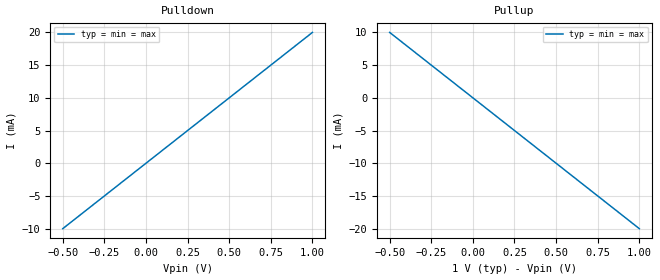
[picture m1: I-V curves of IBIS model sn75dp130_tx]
[IBIS Ver]   5.0
[File Name]  sn75dp130.ibs
[File Rev]   1.0
[Component]  sn75dp130
[Manufacturer] Texas Instruments Incorporated
[Package]
R_pkg  0.0   NA   NA
L_pkg  0.0   NA   NA
C_pkg  0.0   NA   NA
[Pin]   signal_name   model_name   R_pin L_pin  C_pin
1p   Tx_p   sn75dp130_tx
1n   Tx_n   sn75dp130_tx
2p   Rx_p   sn75dp130_rx
2n   Rx_n   sn75dp130_rx
[Diff_Pin] inv_pin vdiff tdelay_typ tdelay_min tdelay_max
2p   2n   NA   NA   NA   NA
1p   1n   NA   NA   NA   NA
[Repeater Pin]
2p 1p
[Model] sn75dp130_rx
Model_type Input
C_comp 0p 0p 0p
Vinl = 0.3
Vinh = 0.7
[Temperature_Range] 25 125 0
[Voltage Range] 1.0 1.0 1.0
[Algorithmic Model]
|Executable Windows_VisualC++ExpressEdition9.0.30729_32 IdealRx.dll IdealRx.ami
Executable Windows_cl15.00.30729.01_32 RX_SN75DP130.dll RX_SN75DP130.ami
[End Algorithmic Model]
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| Models and submodels in the file (2): sn75dp130_tx (Output), sn75dp130_rx (Input)
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[Model] sn75dp130_tx
Model_type Output
C_comp 0p 0p 0p
Cref = 0
Vref = 0.5
Rref = 50
Vmeas = 0.5
[Temperature_Range] 25 125 0
[Voltage Range] 1 1 1
[Algorithmic Model]
|Executable Windows_VisualC++ExpressEdition9.0.30729_32 IdealTx.dll IdealTx.ami
Executable Windows_cl15.00.30729.01_32 TX_SN75DP130.dll TX_SN75DP130.ami
[End Algorithmic Model]
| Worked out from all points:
|   slope of the pulldown table from 0 to 0.15 V, typ, clamps not added: 50 ohm
|   slope of the pullup table from 0 to 0.15 V, typ, clamps not added: 50 ohm
[Pulldown]
-500mV    -10mA      -10mA      -10mA
0V        0A         0A         0A
1V        20mA       20mA       20mA
[Pullup]
-500mV    10mA       10mA       10mA
0V        0A         0A         0A
1V        -20mA      -20mA      -20mA
[GND Clamp]
-500mV    0A         0A         0A
0V        0A         0A         0A
1V        0A         0A         0A
[Power Clamp]
-500mV    0A         0A         0A
0V        0A         0A         0A
1V        0A         0A         0A
[Ramp]
dV/dt_r 0.3/3p 0.3/3p 0.3/3p
dV/dt_f 0.3/3p 0.3/3p 0.3/3p
